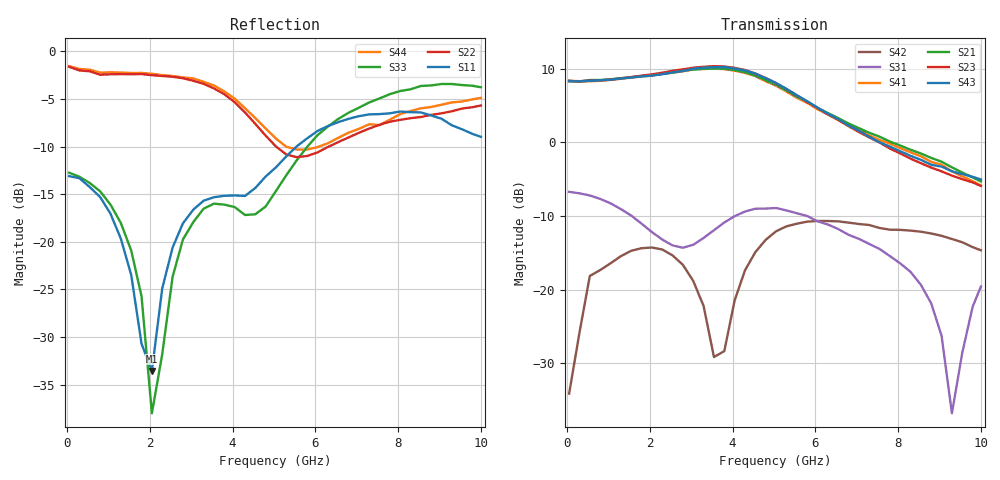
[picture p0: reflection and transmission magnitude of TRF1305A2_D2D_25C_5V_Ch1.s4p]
!Created with skrf (http://scikit-rf.org).
# Hz S MA R 50.0
! PORT[1] = INP
! PORT[2] = OUTM
! PORT[3] = INM
! PORT[4] = OUTP
!freq magS11 angS11 magS12 angS12 magS13 angS13
! magS14 angS14
! magS21 angS21 magS22 angS22 magS23 angS23
! magS24 angS24
! magS31 angS31 magS32 angS32 magS33 angS33
! magS34 angS34
! magS41 angS41 magS42 angS42 magS43 angS43
! magS44 angS44
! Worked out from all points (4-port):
!   41 points, 50 MHz to 10 GHz, reference 50 ohm
!   strongest paths, dB at 50 MHz, 2.55 GHz, 5.05 GHz, 7.55 GHz, 10 GHz:
!     S43: 8.3, 9.5, 8.0, 0.0, -5.1
!     S23: 8.3, 9.7, 8.0, 0.0, -5.9
!     S21: 8.3, 9.5, 7.8, 0.8, -5.3
!     S41: 8.3, 9.4, 7.7, 0.3, -5.9
!     S31: -6.7, -14.0, -8.9, -14.5, -19.6
!     S42: -34.1, -15.4, -12.1, -11.6, -14.7
!   lowest |S11| = -33.5 dB at 2.05 GHz (marker M1), VSWR 1.04, Z = 51.5 + j1.47 ohm
!   |S11| at or under -10 dB: start of sweep to 5.545 GHz
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5e7  0.2212 -1.9  0.004498 15.0  0.4725 -2.5  0.001445 106.9
     2.61 177.6  0.8289 177.5  2.607 -2.5  0.02167 122.1
     0.4604 -2.3  0.002183 152.2  0.2306 -2.6  0.00102 82.2
     2.594 -2.3  0.01968 131.7  2.591 177.4  0.8354 177.8
2.05e9  0.02103 42.8  0.03851 -25.3  0.2449 -111.5  0.02456 -51.2
        2.849 75.6  0.7487 109.7  2.886 -101.0  0.1935 -4.0
        0.2457 -108.8  0.02596 -45.4  0.01259 -84.8  0.03644 -23.1
        2.832 -104.0  0.193 -5.4  2.829 76.4  0.762 108.3
3.3e9  0.1644 44.3  0.05009 -71.8  0.2211 131.6  0.02408 -119.4
       3.145 3.2  0.6748 67.0  3.25 -173.3  0.08146 -66.6
       0.2241 136.0  0.02787 -115.7  0.1492 32.5  0.0479 -69.1
       3.14 -177.0  0.07735 -76.1  3.201 4.6  0.6917 67.1
4.55e9  0.1917 40.1  0.0576 -123.1  0.3414 55.6  0.0185 175.1
        2.828 -79.6  0.4158 32.4  2.923 102.9  0.1707 68.8
        0.3539 57.1  0.0185 178.3  0.1395 21.2  0.05575 -121.6
        2.808 99.1  0.1795 70.3  2.922 -79.4  0.4462 32.0
5.8e9  0.349 23.6  0.05516 -171.5  0.3045 11.1  0.01064 132.6
       1.879 -153.7  0.2821 44.2  1.878 26.6  0.2865 16.7
       0.316 10.6  0.008736 163.3  0.3146 19.4  0.05474 -171.9
       1.852 23.7  0.289 17.5  1.901 -155.7  0.305 40.2
7.55e9  0.4681 -32.2  0.0549 130.2  0.1902 -18.6  0.01132 112.8
        1.09 123.0  0.4113 38.5  0.9958 -57.2  0.2624 -27.1
        0.1887 -17.9  0.0129 140.3  0.5656 -31.6  0.05309 128.1
        1.036 -61.6  0.2619 -23.9  1.001 122.4  0.4101 34.2
1e10  0.3557 -154.7  0.04925 28.0  0.1008 85.6  0.01328 -11.3
      0.5417 14.9  0.5195 3.1  0.5049 -156.5  0.1557 -64.4
      0.1049 86.4  0.01609 29.9  0.6473 -109.1  0.04957 37.5
      0.5087 -174.7  0.1849 -62.7  0.5587 25.1  0.5695 -1.2
